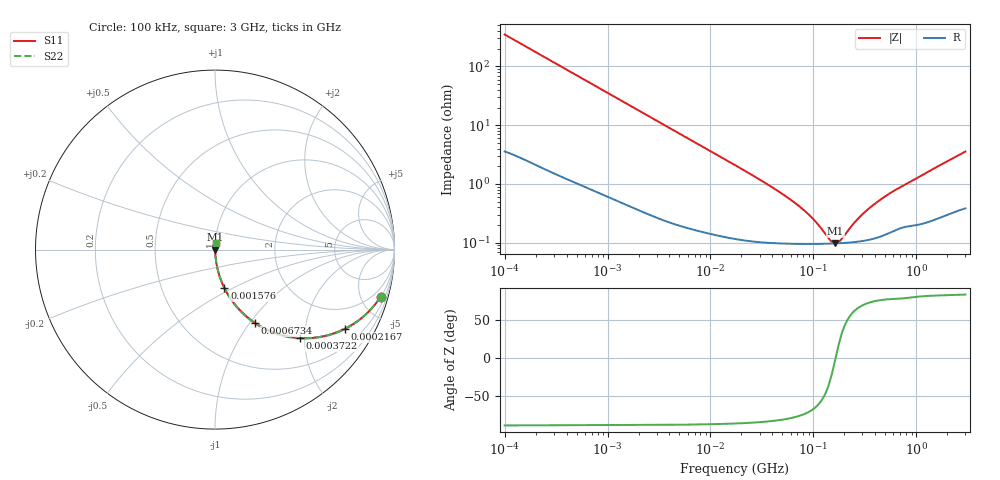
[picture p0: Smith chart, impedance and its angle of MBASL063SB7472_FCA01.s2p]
! MBASL063SB7472_FCA01  S-PARAMETER MODEL  ( Standard Model )
! Model Generated by TAIYO YUDEN Corporation (http://www.ty-top.com)
! Version 1.0
! TAIYO YUDEN Control No. 220601
! Copyright(c) 2020 TAIYO YUDEN CO.,LTD. All Rights Reserved.
! Product Description (link to TY-COMPAS)
! https://ds.yuden.co.jp/TYCOMPAS/or/detail?pn=MBASL063SB7472KFCA01&u=M
! Products Name : Multilayer Ceramic Capacitors
! Characteristics :
!  Capacitance : 4700 [pF] , Rated Voltage : 10 [V] , TCC : X7R
!  Case Size : 0.6 x 0.3 / 0.024 x 0.012 [mm/inch] , Thickness : 0.3 / 0.012 [mm/inch]
!  (Conditions: Temperature = 25 [degC] , DC Bias Voltage = 0 [V])
! External Node Assignments :
!  1  o---| |---o  2
! GND o---------o GND
! Frequency Range : 100kHz  -  3GHz  [ 401 STEP ]
# MHZ S RI R 50
! Freq[MHz].  S11 Real  S11 Imag  S21 Real  S21 Imag  S12 Real  S12 Imag  S22 Real  S22 Imag
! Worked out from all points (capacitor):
!   401 points, 100 kHz to 3 GHz, reference 50 ohm
!   read as one part in series: C = 4.53 nF near 105.3 kHz
!   lowest |Z| = 97.4 mohm at 163.1 MHz (marker M1)
!   series resonance near 164.5 MHz, so ESL is about 210 pH
!   S11 on the Smith chart (normalised r, x): 100 kHz: 1.07, -7.01; 216.7 kHz: 1.04, -3.25; 372.2 kHz: 1.03, -1.90; 673.4 kHz: 1.02, -1.06; 1.576 MHz: 1.01, -0.46; 3 GHz: 1.01, +0.07
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0.1  0.9224 -0.2625  0.0776 0.2625  0.0776 0.2625  0.9224 -0.2625
0.147195  0.848 -0.3534  0.152 0.3534  0.152 0.3534  0.848 -0.3534
0.216663  0.7234 -0.4413  0.2766 0.4413  0.2766 0.4413  0.7234 -0.4413
0.287677  0.6001 -0.4835  0.3999 0.4835  0.3999 0.4835  0.6001 -0.4835
0.372249  0.4752 -0.4927  0.5248 0.4927  0.5248 0.4927  0.4752 -0.4927
0.562235  0.2881 -0.4455  0.7119 0.4455  0.7119 0.4455  0.2881 -0.4455
0.673391  0.2218 -0.4078  0.7782 0.4078  0.7782 0.4078  0.2218 -0.4078
0.991196  0.119 -0.3155  0.881 0.3155  0.881 0.3155  0.119 -0.3155
1.576268  0.0529 -0.2146  0.9471 0.2146  0.9471 0.2146  0.0529 -0.2146
3.161081  0.0154 -0.1122  0.9846 0.1122  0.9846 0.1122  0.0154 -0.1122
6.674626  0.00462 -0.0541  0.9954 0.0541  0.9954 0.0541  0.00462 -0.0541
17.7727  0.00156 -0.0204  0.9984 0.0204  0.9984 0.0204  0.00156 -0.0204
52.46276  0.00101 -0.00631  0.999 0.00631  0.999 0.00631  0.00101 -0.00631
73.34282  0.000972 -0.00403  0.999 0.00403  0.999 0.00403  0.000972 -0.00403
97.38194  0.00096 -0.00246  0.999 0.00246  0.999 0.00246  0.00096 -0.00246
147.0833  0.000967 -0.000503  0.999 0.000503  0.999 0.000503  0.000967 -0.000503
163.0551  0.000973 -3.98e-05  0.999 3.98e-05  0.999 3.98e-05  0.000973 -3.98e-05
185.4806  0.000984 0.000539  0.999 -0.000539  0.999 -0.000539  0.000984 0.000539
246.2744  0.00103 0.00186  0.999 -0.00186  0.999 -0.00186  0.00103 0.00186
310.5665  0.00109 0.00304  0.9989 -0.00304  0.9989 -0.00304  0.00109 0.00304
547.5153  0.00151 0.00667  0.9985 -0.00667  0.9985 -0.00667  0.00151 0.00667
3000  0.00506 0.0351  0.9949 -0.0351  0.9949 -0.0351  0.00506 0.0351
